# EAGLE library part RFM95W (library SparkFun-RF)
RFM95/96/97/98 The RFM95/96/97/98(W) transceivers feature the LoRaTM long range modem that provides ultra-long range spread spectrum communication and high interference immunity whilst minimising current consumption. These devices also support high performance (G)FSK modes for systems including WMBus, IEEE802.15.4g. The RFM95/96/97/98(W) deliver exceptional phase noise, selectivity, receiver linearity and IIP3 for significantly lower current consumption than competing devices Datasheet
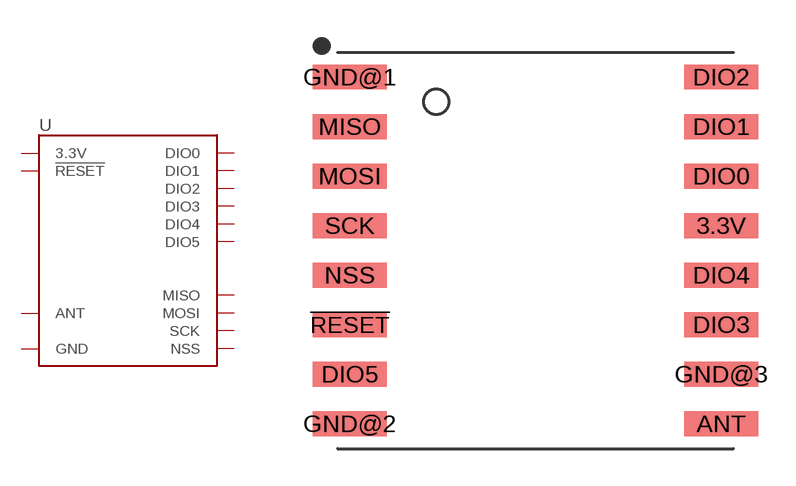
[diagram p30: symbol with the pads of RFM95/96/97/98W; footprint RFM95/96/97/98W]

Designator prefix U

## RFM95W (PROD_ID: IC-13959)  [RFM95/96/97/98W]
3.3V  3.3V
!RESET  !RESET
ANT  ANT
DIO0  DIO0
DIO1  DIO1
DIO2  DIO2
DIO3  DIO3
DIO4  DIO4
DIO5  DIO5
GND@1  GND
GND@2  GND
GND@3  GND
MISO  MISO
MOSI  MOSI
NSS  NSS
SCK  SCK

## Footprint RFM95/96/97/98W (pad centres in mm)
RFM95/96/97/98 The RFM95/96/97/98(W) transceivers feature the LoRaTM long range modem that provides ultra-long range spread spectrum communication and high interference immunity whilst minimising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
smd 3 x 1: 3.3V 7.5,1; !RESET -7.5,-3; ANT 7.5,-7; DIO0 7.5,3; DIO1 7.5,5; DIO2 7.5,7; DIO3 7.5,-3; DIO4 7.5,-1; DIO5 -7.5,-5; GND@1 -7.5,7; GND@2 -7.5,-7; GND@3 7.5,-5; MISO -7.5,5; MOSI -7.5,3; NSS -7.5,-1; SCK -7.5,1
